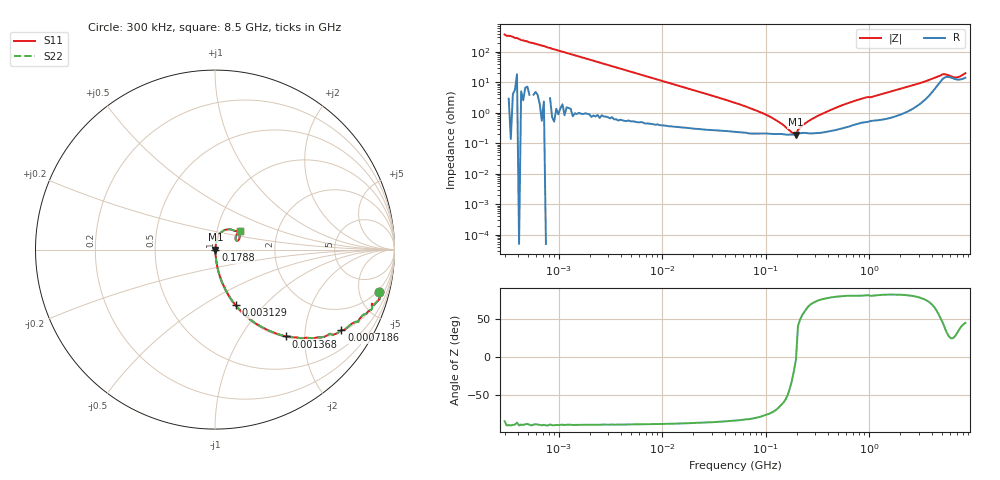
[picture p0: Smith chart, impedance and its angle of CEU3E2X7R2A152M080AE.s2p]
! S-parameter Generated by TDK Corporation
! Copyright(C) 2015 TDK Corporation.
! All Rights Reserved.
! TDK P/N: CEU3E2X7R2A152M080AE (Multilayer Ceramic Chip Capacitors)
! Property: C=1.5nF
! Size(LxWxT): 1.6x0.8x0.8mm, 0.063x0.031x0.031inches
! Model Type: s2p (Touchstone File Format Version 1.0)
! Frequency: DC=Yes Start=0.3MHz Stop=8500MHz 225points Log-sweep
! Note:
! Model Generated on Jun. 23, 2015
! Hash(MD5):
! Port Assignments:
!  1 ---| |--- 2
! Applicable Conditions:
!  Temperature = 25 degC
!  DC Bias Voltage = 0 V
!  Small Signal Operation
! Terms and conditions regarding TDK Simulation Models
! (1)This simulation model is being provided solely for informational purposes. Please refer to the specifications of the products in terms of detailed characteristics of such products.
! (2)In no event shall TDK Corporation of any of its subsidiaries be liable for any loss or damage arising, directly or indirectly,
!  From any information contained in this simulation model, including, but not limited to loss or damages arising from any inaccuracies, omissions or errors in connection with such information.
! (3)Any and all copyrights on this simulation model are owned by TDK Corporation.
!  Duplication or redistribution of this simulation model without prior written permission from TDK Corporation is prohibited.
! (4)This simulation model is subject to any modification or change without any prior notice.
! (5)Neither TDK Corporation nor any of its subsidiaries shall make any warranty, express or implied,
!  Including but not limited to the correctness, implied warranties of merchantability and fitness for a particular purpose with respect to this simulation models.
! (6)The use of this simulation model shall be deemed to have consented to the terms and conditions hereof.
# MHz S MA R 50
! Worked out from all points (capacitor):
!   224 points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, 300 kHz to 8.5 GHz, reference 50 ohm
!   read as one part in series: C = 1.46 nF near 314.1 kHz
!   lowest |Z| = 194 mohm at 196 MHz (marker M1)
!   series resonance near 196.5 MHz, so ESL is about 450 pH
!   S11 on the Smith chart (normalised r, x): 300 kHz: 1.73, -7.41; 718.6 kHz: 1.05, -3.11; 1.368 MHz: 1.02, -1.61; 3.129 MHz: 1.01, -0.71; 178.8 MHz: 1.00, -0.00; 8.5 GHz: 1.28, +0.28
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0.3  0.943 -14.6  0.2532 69.8  0.2532 69.8  0.943 -14.6
0.3141136  0.9583 -16.6  0.2858 73.4  0.2858 73.4  0.9583 -16.6
0.4138848  0.9354 -20.7  0.3536 69.3  0.3536 69.3  0.9354 -20.7
0.7185633  0.8351 -32.5  0.5375 56.6  0.5375 56.6  0.8351 -32.5
1.36767  0.6239 -50.9  0.7756 38.6  0.7756 38.6  0.6239 -50.9
1.72111  0.537 -56.7  0.836 32.5  0.836 32.5  0.537 -56.7
3.12867  0.3315 -69.6  0.9373 19.4  0.9373 19.4  0.3315 -69.6
9.430415  0.1173 -81.4  0.9892 6.7  0.9892 6.7  0.1173 -81.4
51.67171  0.02072 -82.3  0.9974 1.2  0.9974 1.2  0.02072 -82.3
107.8202  0.007747 -74.2  0.9979 0.4  0.9979 0.4  0.007747 -74.2
142.0669  0.004393 -62.4  0.998 0.2  0.998 0.2  0.004393 -62.4
178.7805  0.00227 -31.5  0.9981 0.1  0.9981 0.1  0.00227 -31.5
195.9978  0.001932 -3.2  0.9981 0.0  0.9981 0.0  0.001932 -3.2
205.2186  0.002784 40.9  0.9979 -0.1  0.9979 -0.1  0.002784 40.9
224.9819  0.003788 54.8  0.9978 -0.2  0.9978 -0.2  0.003788 54.8
283.1228  0.006399 70.4  0.9979 -0.3  0.9979 -0.3  0.006399 70.4
590.7752  0.01942 79.3  0.9966 -1.1  0.9966 -1.1  0.01942 79.3
1551.304  0.04787 79.4  0.9923 -2.7  0.9923 -2.7  0.04787 79.4
3548.748  0.1068 68.8  0.9666 -5.9  0.9666 -5.9  0.1068 68.8
5126.239  0.1623 38.8  0.8795 -6.6  0.8795 -6.6  0.1623 38.8
6754.475  0.1279 24.1  0.8847 -3.4  0.8847 -3.4  0.1279 24.1
8500  0.1737 37.8  0.8692 -7.0  0.8692 -7.0  0.1737 37.8
